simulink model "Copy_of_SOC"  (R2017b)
settings: Solver=FixedStepDiscrete  StartTime=0.0  StopTime=10.0  FixedStep=0.01  RelTol=1e-3  EnableMultiTasking=on
undefined symbols (not defined in the file): ASWTYPE_FALSE, ASWTYPE_TRUE, CaSOC_OneSOCVoltTable_mV, CaSOC_ZeroSOCTempTable_C, CaSOC_ZeroSOCVoltTable_mV, CbSOC_ManualDeplaCorrect_flg, CbSOC_ManuOCVCorrect_flg, CbSOC_SOCHighDiagOn_flg, CbSOC_SOCLowDiagOn_flg, CcSOC_ACChrgFinishDispSOC_pct, CcSOC_ACChrgFinishMaxSOC_pct, CcSOC_ACStepChrgMaxSOC_pct, CcSOC_AllowMaxCellSOC_pct, CcSOC_AllowMinCellSOC_pct, CcSOC_CapCalcCycl_ms, CcSOC_CellMinTempFilterAvg_numb, CcSOC_CellVoltMeasTol_mV, CcSOC_ChrgFishBefMaxSOC_pct, CcSOC_ChrgFishBefMinSOC_pct, CcSOC_ChrgFollowCurr_A, CcSOC_DCChrgFinishDispSOC_pct, CcSOC_DCChrgFinishMaxSOC_pct, CcSOC_DCStepChrgMaxSOC_pct, CcSOC_DeplaCellVoltMeasTol_mV, CcSOC_DeplaCorrectSOCDiff_pct, CcSOC_DisChrgFlwCurr_A, CcSOC_DispSOCChgSleepTime_min, CcSOC_DispSOCCordRunTi_ms, CcSOC_DispSOCErr_pct, CcSOC_FlwTarSOCDiff_pct, CcSOC_FullChrgTempThrld_C, CcSOC_MaxFlwDispSOC_pct, CcSOC_MinFlwDispSOC_pct, CcSOC_OCVCorrectRunTime_ms, CcSOC_OCVCorrectSleepTime_min, CcSOC_OCVCorrectSOCDiff_pct, CcSOC_OCVPeakCellVoltDev_mV, CcSOC_OCVPeakCellVoltTime_ms, CcSOC_PackSOCUseMax_pct, CcSOC_PackSOCUseMin_pct, CcSOC_SOCDeplaCurrThrd_A, CcSOC_SOCDeplaCurrThrdTi_ms, CcSOC_SOCDeplaNoOCVTi_min, CcSOC_SOCDeplaOCVTi_min, CcSOC_SOCHighAlarmThrld_pct, CcSOC_SOCHighWarningThrld_pct, CcSOC_SOCHysValue_pct, CcSOC_SOCLowAlarmThrld_pct, CcSOC_SOCLowWarningThrld_pct, CcSOC_ZeroMinSOC_pct, CcSOC_ZeroPackCrntThrd_A, CcSOC_ZeroSOCRunTime_ms, Enum_CTCCtrCtlConnMode, Enum_MSMBMUState, SOC_CONST0_NUMB, SOC_CONST1000_NUMB, SOC_CONST100_NUMB, SOC_CONST2080_NUMB, SOC_CONST3600000_NUMB, SOC_CONST60000_NUMB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
libraries: AIWAYS_Powertrain_BMS_lib x109
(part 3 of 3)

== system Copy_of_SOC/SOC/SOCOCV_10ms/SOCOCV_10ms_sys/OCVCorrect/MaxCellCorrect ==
  LcSOC_OCVSOCMaxSOC_pct : Inport
  LcSOC_OCVSOCMinSOC_pct : Inport  Port=2
  GcCDP_MaxCellVolt_mV : Inport  Port=3
  GcCDP_MinCellVolt_mV : Inport  Port=4
  Enable : EnablePort
  Data Store Write : AIWAYS_Powertrain_BMS_lib/Signals/Data Store Write  DSW=EcNVM_MaxCellSOC_pct
  Data Store Write1 : AIWAYS_Powertrain_BMS_lib/Signals/Data Store Write  DSW=EcNVM_MinCellSOC_pct
  Data Store Write2 : AIWAYS_Powertrain_BMS_lib/Signals/Data Store Write  DSW=EcNVM_SOCCorrdMaxCellVolt_mV
  Data Store Write3 : AIWAYS_Powertrain_BMS_lib/Signals/Data Store Write  DSW=EcNVM_SOCCorrdMinCellVolt_mV
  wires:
  LcSOC_OCVSOCMinSOC_pct/1 -> Data Store Write1/1
  LcSOC_OCVSOCMaxSOC_pct/1 -> Data Store Write/1
  GcCDP_MinCellVolt_mV/1 -> Data Store Write3/1
  GcCDP_MaxCellVolt_mV/1 -> Data Store Write2/1

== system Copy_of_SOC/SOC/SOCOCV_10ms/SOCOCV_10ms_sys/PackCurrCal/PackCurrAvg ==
  LcSOC_SumPackCurr_A : Inport
  Enable : EnablePort
  Constant4 : Constant  Value=SOC_RUNTIME_MS
  Constant5 : Constant  Value=CcSOC_CapCalcCycl_ms
  Divide : Product  Inputs=*/  OutDataTypeStr=Inherit: Inherit via back propagation  RndMeth=Round
  Divide1 : Product  Inputs=*/  OutDataTypeStr=uint8  RndMeth=Round
  LcSOC_PackCurrAvg_A : Outport
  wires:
  LcSOC_SumPackCurr_A/1 -> Divide/1
  Divide1/1 -> Divide/2
  Constant4/1 -> Divide1/2
  Divide/1 -> LcSOC_PackCurrAvg_A/1  "LcSOC_PackCurrAvg_A"
  Constant5/1 -> Divide1/1

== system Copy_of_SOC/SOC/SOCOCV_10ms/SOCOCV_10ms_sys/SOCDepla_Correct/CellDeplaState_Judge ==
  GcCDP_MaxCellVolt_mV : Inport
  GcCDP_MinCellVolt_mV : Inport  Port=2
  GbCDP_SumCellVoltVld_flg : Inport  Port=3
  Enable : EnablePort  StatesWhenEnabling=reset
  Add : Sum  Inputs=+-  OutDataTypeStr=single
  Add1 : Sum  OutDataTypeStr=single
  Constant : Constant  Value=CcSOC_DeplaCellVoltMeasTol_mV
  Constant1 : Constant  Value=ASWTYPE_FALSE
  Constant11 : Constant  Value=ASWTYPE_FALSE
  Data Type Conversion : DataTypeConversion  OutDataTypeStr=single
  Data Type Conversion1 : DataTypeConversion  OutDataTypeStr=single
  Demux : Demux  Outputs=2
  Logical Operator : Logic  Inputs=3  AllPortsSameDT=off  OutDataTypeStr=boolean
  Logical Operator2 : Logic  Operator=OR  AllPortsSameDT=off  OutDataTypeStr=boolean
  Mux : Mux  Inputs=2
  Relational Operator : RelationalOperator  OutDataTypeStr=boolean
  Relational Operator1 : RelationalOperator  Operator===  OutDataTypeStr=boolean
  Relational Operator2 : RelationalOperator  Operator===  OutDataTypeStr=boolean
  Unit Delay : UnitDelay  SampleTime=-1  StateName=StateName
  Unit Delay External IC : AIWAYS_Powertrain_BMS_lib/Delay Blocks/Unit Delay External IC
  Unit Delay1 : UnitDelay  SampleTime=-1  StateName=StateName
  LbSOC_DeplaCellVoltChrgState_flg : Outport
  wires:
  GcCDP_MaxCellVolt_mV/1 -> Data Type Conversion/1
  GcCDP_MinCellVolt_mV/1 -> Data Type Conversion1/1
  Mux/1 -> Unit Delay External IC/2, Unit Delay External IC/1, Add/1
  Unit Delay External IC/1 -> Add/2
  Add/1 -> Add1/1
  Unit Delay/1 -> Add1/2
  Add1/1 -> Unit Delay/1, Relational Operator/1
  Constant/1 -> Relational Operator/2
  Relational Operator/1 -> Demux/1
  Demux/1 -> Logical Operator/1
  Demux/2 -> Logical Operator/2
  Logical Operator/1 -> LbSOC_DeplaCellVoltChrgState_flg/1  "LbSOC_DeplaCellVoltChrgState_flg"
  GbCDP_SumCellVoltVld_flg/1 -> Relational Operator2/1
  Constant11/1 -> Relational Operator2/2
  Unit Delay1/1 -> Logical Operator2/2
  Logical Operator2/1 -> Relational Operator1/1, Unit Delay1/1
  Relational Operator2/1 -> Logical Operator2/1
  Constant1/1 -> Relational Operator1/2
  Relational Operator1/1 -> Logical Operator/3
  Data Type Conversion/1 -> Mux/1
  Data Type Conversion1/1 -> Mux/2

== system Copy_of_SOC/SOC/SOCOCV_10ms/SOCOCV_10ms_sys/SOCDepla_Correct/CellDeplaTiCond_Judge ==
  GcSOC_CellDeplaTi_min : Inport
  LbSOC_DeplaCellVoltChrgState_flg : Inport  Port=2
  LbSOC_OCVCorrectOn_flg : Inport  Port=3
  GcCDP_MaxCellVolt_mV : Inport  Port=4
  GcCDP_MinCellVolt_mV : Inport  Port=5
  GbCDP_SumCellVoltVld_flg : Inport  Port=6
  GeUDS_CapSel_enum : Inport  Port=7
  Bus Creator : BusCreator  Inputs=4
  Bus Selector : BusSelector  OutputSignals=GcSOC_CellDeplaTi_min,LbSOC_OCVCorrectOn_flg
  Bus Selector1 : BusSelector  OutputSignals=GcSOC_CellDeplaTi_min,LbSOC_OCVCorrectOn_flg
  Bus Selector6 : BusSelector  OutputSignals=GcCDP_MaxCellVolt_mV,GcCDP_MinCellVolt_mV
  Constant1 : Constant  Value=CbSOC_ManualDeplaCorrect_flg
  Constant6 : Constant  Value=CcSOC_SOCDeplaOCVTi_min
  Constant7 : Constant  Value=CcSOC_SOCDeplaNoOCVTi_min
  Constant9 : Constant  Value=ASWTYPE_FALSE
  EdgeRising : AIWAYS_Powertrain_BMS_lib/Logical Operators/EdgeRising
  Logical Operator5 : Logic  Inputs=3  AllPortsSameDT=off  OutDataTypeStr=boolean
  Logical Operator6 : Logic  Inputs=3  AllPortsSameDT=off  OutDataTypeStr=boolean
  Logical Operator7 : Logic  Operator=OR  AllPortsSameDT=off  OutDataTypeStr=boolean
  Logical Operator8 : Logic  AllPortsSameDT=off  OutDataTypeStr=boolean
  Relational Operator3 : RelationalOperator  OutDataTypeStr=boolean
  Relational Operator4 : RelationalOperator  Operator===  OutDataTypeStr=boolean
  Relational Operator5 : RelationalOperator  OutDataTypeStr=boolean
  SOCDepla_Correct2 : Subsystem  TreatAsAtomicUnit=on
  SOC_GbSOC_SOCDeplaTiReach_flg : AIWAYS_Powertrain_BMS_lib/Signals/OverWrite  OverWrite_Value=CbSOC_SOCDeplaTiReachOvr_flg  OverWrite_flag=CbSOC_SOCDeplaTiReachOvrSwt_flg
  GbSOC_SOCDeplaTiReach_flg : Outport
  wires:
  Bus Selector6/1 -> SOCDepla_Correct2/2(GcCDP_MaxCellVolt_mV)  "<GcCDP_MaxCellVolt_mV>"
  Bus Selector6/2 -> SOCDepla_Correct2/3(GcCDP_MinCellVolt_mV)  "<GcCDP_MinCellVolt_mV>"
  Constant6/1 -> Relational Operator3/2
  Relational Operator3/1 -> Logical Operator5/2
  Logical Operator5/1 -> Logical Operator7/2  "LbSOC_SOCDeplaOCV_flg"
  Relational Operator5/1 -> Logical Operator6/1
  Constant7/1 -> Relational Operator5/2
  Bus Creator/1 -> Bus Selector/1, Bus Selector1/1, Bus Selector6/1
  Bus Selector/1 -> Relational Operator5/1  "<GcSOC_CellDeplaTi_min>"
  Constant9/1 -> Relational Operator4/2
  Relational Operator4/1 -> Logical Operator6/2
  Bus Selector/2 -> Relational Operator4/1  "<LbSOC_OCVCorrectOn_flg>"
  Bus Selector1/1 -> Relational Operator3/1  "<GcSOC_CellDeplaTi_min>"
  Bus Selector1/2 -> Logical Operator5/3  "<LbSOC_OCVCorrectOn_flg>"
  Logical Operator6/1 -> Logical Operator7/1  "LbSOC_SOCDeplaNoOCV_flg"
  LbSOC_DeplaCellVoltChrgState_flg/1 -> SOCDepla_Correct2/1(LbSOC_DeplaCellVoltChrgState_flg)
  EdgeRising/1 -> SOCDepla_Correct2/Enable
  Logical Operator8/1 -> SOC_GbSOC_SOCDeplaTiReach_flg/1
  GcSOC_CellDeplaTi_min/1 -> Bus Creator/1
  GcCDP_MinCellVolt_mV/1 -> Bus Creator/4
  GcCDP_MaxCellVolt_mV/1 -> Bus Creator/3
  LbSOC_OCVCorrectOn_flg/1 -> Bus Creator/2
  Logical Operator7/1 -> Logical Operator8/2
  GbCDP_SumCellVoltVld_flg/1 -> Logical Operator8/1
  Constant1/1 -> Logical Operator6/3, Logical Operator5/1
  SOC_GbSOC_SOCDeplaTiReach_flg/1 -> EdgeRising/1, GbSOC_SOCDeplaTiReach_flg/1  "GbSOC_SOCDeplaTiReach_flg"
  GeUDS_CapSel_enum/1 -> SOCDepla_Correct2/4(GeUDS_CapSel_enum)

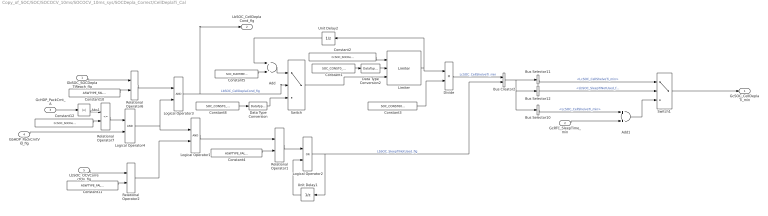
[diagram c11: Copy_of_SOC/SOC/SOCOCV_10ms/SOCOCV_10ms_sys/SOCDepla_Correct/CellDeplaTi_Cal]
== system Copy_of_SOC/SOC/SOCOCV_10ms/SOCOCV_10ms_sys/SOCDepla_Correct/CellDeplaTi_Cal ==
  GbSOC_SOCDeplaTiReach_flg : Inport
  GcRTC_SleepTime_min : Inport  Port=2
  GcHDP_PackCrnt_A : Inport  Port=3
  GbHDP_PackCrntVld_flg : Inport  Port=4
  LbSOC_OCVCorrectOn_flg : Inport  Port=5
  Abs1 : Abs
  Add : Sum  OutDataTypeStr=uint32
  Add1 : Sum  OutDataTypeStr=uint32
  Bus Creator2 : BusCreator  Inputs=2
  Bus Selector10 : BusSelector  OutputSignals=LcSOC_CellShelveTi_min
  Bus Selector11 : BusSelector  OutputSignals=LcSOC_CellShelveTi_min
  Bus Selector12 : BusSelector  OutputSignals=LbSOC_SleepTiNotUsed_flg
  Constant1 : Constant  Value=SOC_CONST0_NUMB
  Constant10 : Constant  Value=ASWTYPE_FALSE
  Constant11 : Constant  Value=ASWTYPE_FALSE
  Constant12 : Constant  Value=CcSOC_SOCDeplaCurrThrd_A
  Constant2 : Constant  Value=CcSOC_SOCDeplaCurrThrdTi_ms
  Constant3 : Constant  Value=SOC_CONST60000_NUMB
  Constant4 : Constant  Value=ASWTYPE_FALSE
  Constant5 : Constant  Value=SOC_RUNTIME_MS
  Constant8 : Constant  Value=SOC_CONST0_NUMB
  Data Type Conversion : DataTypeConversion
  Data Type Conversion2 : DataTypeConversion
  Divide : Product  Inputs=*/  OutDataTypeStr=Inherit: Inherit via back propagation  RndMeth=Round
  Limiter : AIWAYS_Powertrain_BMS_lib/Nonlinear Blocks/Limiter
  Logical Operator1 : Logic  AllPortsSameDT=off  OutDataTypeStr=boolean
  Logical Operator2 : Logic  Operator=OR  AllPortsSameDT=off  OutDataTypeStr=boolean
  Logical Operator3 : Logic  AllPortsSameDT=off  OutDataTypeStr=boolean
  Logical Operator4 : Logic  AllPortsSameDT=off  OutDataTypeStr=boolean
  Relational Operator1 : RelationalOperator  Operator===  OutDataTypeStr=boolean
  Relational Operator2 : RelationalOperator  Operator===  OutDataTypeStr=boolean
  Relational Operator6 : RelationalOperator  Operator===  OutDataTypeStr=boolean
  Relational Operator7 : RelationalOperator  Operator=<=  OutDataTypeStr=boolean
  Switch : Switch  Criteria=u2 ~= 0
  Switch1 : Switch  Criteria=u2 ~= 0
  Unit Delay1 : UnitDelay  SampleTime=-1  StateName=StateName
  Unit Delay2 : UnitDelay  SampleTime=-1  StateName=StateName
  GcSOC_CellDeplaTi_min : Outport
  LbSOC_CellDeplaCond_flg : Outport  Port=2
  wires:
  Divide/1 -> Bus Creator2/1  "LcSOC_CellShelveTi_min"
  Constant5/1 -> Add/2
  Add/1 -> Switch/1
  Switch/1 -> Limiter/3
  Constant1/1 -> Data Type Conversion2/1
  Constant2/1 -> Limiter/1
  Limiter/1 -> Unit Delay2/1, Divide/1
  Constant3/1 -> Divide/2
  Add1/1 -> Switch1/3
  GcRTC_SleepTime_min/1 -> Add1/2
  Switch1/1 -> GcSOC_CellDeplaTi_min/1
  Logical Operator3/1 -> LbSOC_CellDeplaCond_flg/1, Switch/2  "LbSOC_CellDeplaCond_flg"
  Unit Delay2/1 -> Add/1
  Constant10/1 -> Relational Operator6/2
  Relational Operator6/1 -> Logical Operator3/1
  Relational Operator7/1 -> Logical Operator4/1
  Abs1/1 -> Relational Operator7/1
  Constant12/1 -> Relational Operator7/2
  Bus Selector12/1 -> Switch1/2  "<LbSOC_SleepTiNotUsed_flg>"
  Bus Creator2/1 -> Bus Selector10/1, Bus Selector12/1, Bus Selector11/1
  Bus Selector10/1 -> Add1/1  "<LcSOC_CellShelveTi_min>"
  Bus Selector11/1 -> Switch1/1  "<LcSOC_CellShelveTi_min>"
  GcHDP_PackCrnt_A/1 -> Abs1/1
  GbHDP_PackCrntVld_flg/1 -> Logical Operator4/2
  Logical Operator4/1 -> Logical Operator3/2, Logical Operator1/1
  Relational Operator2/1 -> Logical Operator1/2
  Constant11/1 -> Relational Operator2/2
  Logical Operator1/1 -> Relational Operator1/1
  Constant4/1 -> Relational Operator1/2
  Relational Operator1/1 -> Logical Operator2/1
  Unit Delay1/1 -> Logical Operator2/2
  Logical Operator2/1 -> Bus Creator2/2, Unit Delay1/1  "LbSOC_SleepTiNotUsed_flg"
  LbSOC_OCVCorrectOn_flg/1 -> Relational Operator2/1
  GbSOC_SOCDeplaTiReach_flg/1 -> Relational Operator6/1
  Constant8/1 -> Data Type Conversion/1
  Data Type Conversion/1 -> Switch/3
  Data Type Conversion2/1 -> Limiter/2

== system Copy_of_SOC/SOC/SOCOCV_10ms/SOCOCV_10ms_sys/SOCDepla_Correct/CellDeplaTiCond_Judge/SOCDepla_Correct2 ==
  LbSOC_DeplaCellVoltChrgState_flg : Inport
  GcCDP_MaxCellVolt_mV : Inport  Port=2
  GcCDP_MinCellVolt_mV : Inport  Port=3
  GeUDS_CapSel_enum : Inport  Port=4
  Enable : EnablePort  StatesWhenEnabling=reset
  2D_Config_Word : AIWAYS_Powertrain_BMS_lib/Signals/2D_Config_Word  Default_Cal_Breakpoint1_Name=CaSOC_CATL203ChrgDeplaSOCCellVolt_mV  Default_Cal_Table1_Name=CaSOC_CATL203ChrgDeplaSOCCellSOC_pct  CATL153Ah_Cal_Breakpoint1_Name=CaSOC_TFE177ChrgDeplaSOCCellVolt_mV  CATL153Ah_Cal_Table1_Name=CaSOC_TFE177ChrgDeplaSOCCellSOC_pct  CATL180Ah_Cal_Breakpoint1_Name=CaSOC_TFE177ChrgDeplaSOCCellVolt_mV  CATL180Ah_Cal_Table1_Name=CaSOC_TFE177ChrgDeplaSOCCellSOC_pct  CATL177Ah_Cal_Breakpoint1_Name=CaSOC_CATL177ChrgDeplaSOCCellVolt_mV  CATL177Ah_Cal_Table1_Name=CaSOC_CATL177ChrgDeplaSOCCellSOC_pct  CATL203Ah_Cal_Breakpoint1_Name=CaSOC_CATL203ChrgDeplaSOCCellVolt_mV  CATL203Ah_Cal_Table1_Name=CaSOC_CATL203ChrgDeplaSOCCellSOC_pct  CATL51Ah_Cal_Breakpoint1_Name=CaSOC_TFE177ChrgDeplaSOCCellVolt_mV  CATL51Ah_Cal_Table1_Name=CaSOC_TFE177ChrgDeplaSOCCellSOC_pct  CATL132Ah_Cal_Breakpoint1_Name=CaSOC_TFE177ChrgDeplaSOCCellVolt_mV  CATL132Ah_Cal_Table1_Name=CaSOC_TFE177ChrgDeplaSOCCellSOC_pct  XWD75Ah_Cal_Breakpoint1_Name=CaSOC_XWD75ChrgDeplaSOCCellVolt_mV  XWD75Ah_Cal_Table1_Name=CaSOC_XWD75ChrgDeplaSOCCellSOC_pct  TFE177Ah_Cal_Breakpoint1_Name=CaSOC_TFE177ChrgDeplaSOCCellVolt_mV  TFE177Ah_Cal_Table1_Name=CaSOC_TFE177ChrgDeplaSOCCellSOC_pct  CATLCTP248Ah_Cal_Breakpoint1_Name=CaSOC_TFE177ChrgDeplaSOCCellVolt_mV  CATLCTP248Ah_Cal_Table1_Name=CaSOC_TFE177ChrgDeplaSOCCellSOC_pct
  2D_Config_Word1 : AIWAYS_Powertrain_BMS_lib/Signals/2D_Config_Word  Default_Cal_Breakpoint1_Name=CaSOC_CATL203DisChrgDeplaSOCCellVolt_mV  Default_Cal_Table1_Name=CaSOC_CATL203DisChrgDeplaSOCCellSOC_pct  CATL153Ah_Cal_Breakpoint1_Name=CaSOC_TFE177DisChrgDeplaSOCCellVolt_mV  CATL153Ah_Cal_Table1_Name=CaSOC_TFE177DisChrgDeplaSOCCellSOC_pct  CATL180Ah_Cal_Breakpoint1_Name=CaSOC_TFE177DisChrgDeplaSOCCellVolt_mV  CATL180Ah_Cal_Table1_Name=CaSOC_TFE177DisChrgDeplaSOCCellSOC_pct  CATL177Ah_Cal_Breakpoint1_Name=CaSOC_CATL177DisChrgDeplaSOCCellVolt_mV  CATL177Ah_Cal_Table1_Name=CaSOC_CATL177DisChrgDeplaSOCCellSOC_pct  CATL203Ah_Cal_Breakpoint1_Name=CaSOC_CATL203DisChrgDeplaSOCCellVolt_mV  CATL203Ah_Cal_Table1_Name=CaSOC_CATL203DisChrgDeplaSOCCellSOC_pct  CATL51Ah_Cal_Breakpoint1_Name=CaSOC_TFE177DisChrgDeplaSOCCellVolt_mV  CATL51Ah_Cal_Table1_Name=CaSOC_TFE177DisChrgDeplaSOCCellSOC_pct  CATL132Ah_Cal_Breakpoint1_Name=CaSOC_TFE177DisChrgDeplaSOCCellVolt_mV  CATL132Ah_Cal_Table1_Name=CaSOC_TFE177DisChrgDeplaSOCCellSOC_pct  XWD75Ah_Cal_Breakpoint1_Name=CaSOC_XWD75DisChrgDeplaSOCCellVolt_mV  XWD75Ah_Cal_Table1_Name=CaSOC_XWD75DisChrgDeplaSOCCellSOC_pct  TFE177Ah_Cal_Breakpoint1_Name=CaSOC_TFE177DisChrgDeplaSOCCellVolt_mV  TFE177Ah_Cal_Table1_Name=CaSOC_TFE177DisChrgDeplaSOCCellSOC_pct  CATLCTP248Ah_Cal_Breakpoint1_Name=CaSOC_TFE177DisChrgDeplaSOCCellVolt_mV  CATLCTP248Ah_Cal_Table1_Name=CaSOC_TFE177DisChrgDeplaSOCCellSOC_pct
  Abs : Abs
  Add1 : Sum  Inputs=+-
  Constant : Constant  Value=CcSOC_DeplaCorrectSOCDiff_pct
  Data Store Read2 : AIWAYS_Powertrain_BMS_lib/Signals/Data Store Read  Priority=0  DSR=EcNVM_MaxCellSOC_pct
  Data Store Read3 : AIWAYS_Powertrain_BMS_lib/Signals/Data Store Read  Priority=0  DSR=EcNVM_MinCellSOC_pct
  Demux2 : Demux  Outputs=2
  Logical Operator3 : Logic  Operator=OR  Inputs=1  AllPortsSameDT=off  OutDataTypeStr=boolean
  MaxCellCorrect : Subsystem  TreatAsAtomicUnit=on
  Mux : Mux  Inputs=2
  Mux2 : Mux  Inputs=2
  Relational Operator3 : RelationalOperator  OutDataTypeStr=boolean
  Signal Conversion : SignalConversion  OverrideOpt=off
  Signal Conversion1 : SignalConversion  OverrideOpt=off
  Switch2 : Switch  Criteria=u2 ~= 0
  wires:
  LbSOC_DeplaCellVoltChrgState_flg/1 -> Switch2/2
  GcCDP_MaxCellVolt_mV/1 -> Mux/1
  GcCDP_MinCellVolt_mV/1 -> Mux/2
  Mux/1 -> 2D_Config_Word/2, 2D_Config_Word1/2
  2D_Config_Word/1 -> Switch2/1
  2D_Config_Word1/1 -> Switch2/3
  Add1/1 -> Abs/1
  Relational Operator3/1 -> Logical Operator3/1
  Data Store Read2/1 -> Mux2/1
  Data Store Read3/1 -> Mux2/2
  Abs/1 -> Relational Operator3/1
  Constant/1 -> Relational Operator3/2
  Mux2/1 -> Add1/1
  Signal Conversion/1 -> MaxCellCorrect/1(LcSOC_DeplaSOCMaxSOC_pct)  "LcSOC_DeplaSOCMaxSOC_pct"
  Logical Operator3/1 -> MaxCellCorrect/Enable
  Demux2/1 -> Signal Conversion/1
  Demux2/2 -> Signal Conversion1/1
  Signal Conversion1/1 -> MaxCellCorrect/2(LcSOC_DeplaSOCMinSOC_pct)  "LcSOC_DeplaSOCMinSOC_pct"
  Switch2/1 -> Add1/2, Demux2/1
  GeUDS_CapSel_enum/1 -> 2D_Config_Word1/1, 2D_Config_Word/1

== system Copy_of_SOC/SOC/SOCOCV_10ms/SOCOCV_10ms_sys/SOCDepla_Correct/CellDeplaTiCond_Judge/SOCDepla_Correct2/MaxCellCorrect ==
  LcSOC_DeplaSOCMaxSOC_pct : Inport
  LcSOC_DeplaSOCMinSOC_pct : Inport  Port=2
  Enable : EnablePort  StatesWhenEnabling=reset
  Data Store Write : AIWAYS_Powertrain_BMS_lib/Signals/Data Store Write  DSW=EcNVM_MaxCellSOC_pct
  Data Store Write1 : AIWAYS_Powertrain_BMS_lib/Signals/Data Store Write  DSW=EcNVM_MinCellSOC_pct
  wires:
  LcSOC_DeplaSOCMinSOC_pct/1 -> Data Store Write1/1
  LcSOC_DeplaSOCMaxSOC_pct/1 -> Data Store Write/1

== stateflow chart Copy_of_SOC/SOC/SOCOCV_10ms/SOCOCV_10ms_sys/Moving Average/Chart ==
  (default) -> (junction 16)
  (junction 16) -> (junction 17) : [R]
  (junction 16) -> (junction 18)
  (junction 17) -> (junction 22) : {count = 0;...  sum = 0;...  buffer = 0;...  average = 0;...  index = 0;}
  (junction 18) -> (junction 19) : [count >= BufferSize]
  (junction 18) -> (junction 21) : {count = count +1;}
  (junction 19) -> (junction 20) : {sum = sum - buffer[index];}
  (junction 20) -> (junction 21)
  (junction 21) -> (junction 25) : {sum = sum + u;... buffer[index] =u;... average = sum/count;}
  (junction 25) -> (junction 24) : [index >= BufferSize-1]
  (junction 25) -> (junction 26) : {index = index+1;}
  (junction 24) -> (junction 27) : {index = 0;}
  (junction 27) -> (junction 26)
  (junction 22) -> (junction 27)
  (junction 26) -> (junction 23) : {Y=average;}
  data: count local uint16 [0..500]; buffer local single; u input single; index local uint16 [0..499]; R input boolean; sum local single; BufferSize parameter uint16 [1..500]; Y output single; average local single

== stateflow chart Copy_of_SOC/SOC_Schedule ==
  (default) -> (junction 50)
  (junction 50) -> (junction 13) : { SOC_SOCOCV_10ms; }
  (junction 13) -> (junction 150) : { TimeCounter100ms ++; }
  (junction 150) -> (junction 422) : [TimeCounter100ms >= Const100ms]
  (junction 150) -> (junction 424)
  (junction 422) -> (junction 424) : { SOC_SOCCal_100ms; SOC_SOCDisp_100ms; TimeCounter100ms = 0; }
  data: TimeCounter100ms local uint8; Const100ms constant uint8 =10
  events: output FUNCTION_CALL_EVENT; output FUNCTION_CALL_EVENT; output FUNCTION_CALL_EVENT
